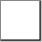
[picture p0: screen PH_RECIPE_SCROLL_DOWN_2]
VISUALIZATION PH_RECIPE_SCROLL_DOWN_2  // 42x42
VAR_IN_OUT
	RECIPE_CTRL_V2 : None;
END_VAR
    Rectangle (0,0 40x40)
        tap RECIPE_CTRL_V2.sCmd.bScrollDown
    Polygon (20,30), colour toggle: (RECIPE_CTRL_V2.sCmd.bScrollDown) <> 0
        tap RECIPE_CTRL_V2.sCmd.bScrollDown
END_VISUALIZATION
